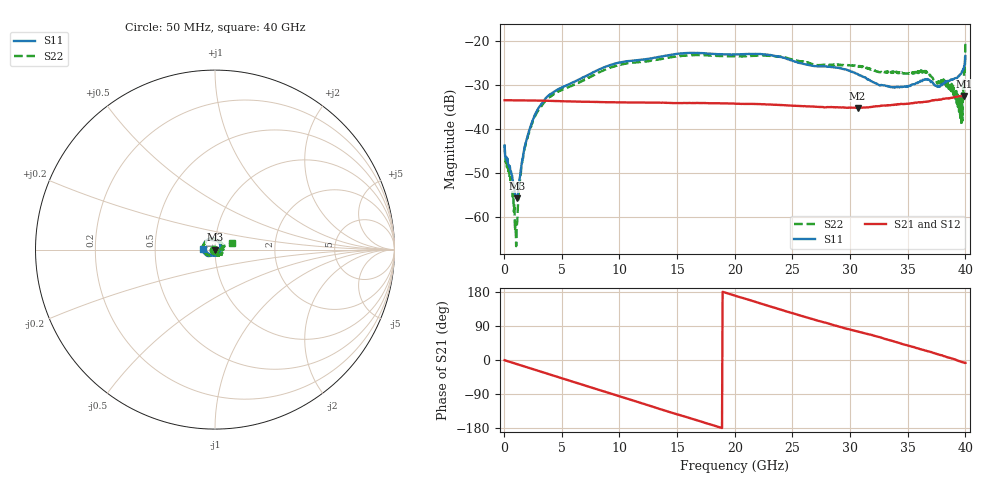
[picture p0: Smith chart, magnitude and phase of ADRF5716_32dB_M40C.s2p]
! Device: ADRF5716
! Description: 30GHz 2-Bit Digital Attenuator
! Frequency: 100 MHz – 30 GHz
! Ports:
! ATTIN  = Port 1
! ATTOUT = Port 2
! State: 32 dB Attenuation selected
! Supply Voltage:
! VDD  =  +3.30 Volts
! VSS  =  -3.30 Volts
! Control Voltages:
! D5 = 0V, D6 = 3.3V
! Temperature = -40 C
! Data: Data was collected using a calibrated network analyzer.
!  The reference plane is the package pins of ADRF5716 switch.
! Note: Analog Devices supplies this data as a sample of measured data for this product.
!  Your particular data for this product may vary.
!  Analog Devices reserves the right to change this data at anytime
# HZ S DB R 50
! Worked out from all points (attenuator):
!   800 points, 50 MHz to 40 GHz, reference 50 ohm
!   highest |S21| = -32.51 dB at 39.9 GHz (marker M1); lowest = -35.2 dB at 30.65 GHz (marker M2)
!   lowest |S11| = -55.8 dB at 1.1 GHz (marker M3), VSWR 1.00, Z = 49.9 - j0.119 ohm
!   |S11| at or under -10 dB: start of sweep to end of sweep
!   |S22| runs from -66.7 to -19.9 dB; largest |S21 - S12| = 0
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5e7  -43.81 -140.6  -33.48 -0.6  -33.48 -0.6  -43.64 -138.2
6e8  -49.65 177.3  -33.49 -5.9  -33.49 -5.9  -50.97 168.2
9.5e8  -54.84 -154.8  -33.51 -9.3  -33.51 -9.3  -63.17 -178.2
1.1e9  -55.77 -132.8  -33.52 -10.7  -33.52 -10.7  -62.14 -112.1
1.5e9  -48.55 -79.6  -33.53 -14.5  -33.53 -14.5  -48.74 -63.2
1.7e9  -45.37 -75.1  -33.53 -16.4  -33.53 -16.4  -45.27 -63.5
2.7e9  -36.64 -83.6  -33.55 -26.0  -33.55 -26.0  -36.96 -79.7
3.9e9  -32.30 -102.0  -33.62 -37.6  -33.62 -37.6  -32.87 -101.0
6.75e9  -28.42 -121.9  -33.81 -64.6  -33.81 -64.6  -29.17 -124.0
9.65e9  -25.12 -141.2  -33.95 -92.4  -33.95 -92.4  -25.67 -144.2
1.34e10  -23.63 -163.8  -34.03 -128.1  -34.03 -128.1  -24.20 -169.7
2.005e10  -23.06 154.0  -34.26 169.5  -34.26 169.5  -23.48 143.9
2.67e10  -25.64 101.0  -34.92 108.3  -34.92 108.3  -25.31 82.9
3.065e10  -27.55 49.6  -35.22 75.2  -35.22 75.2  -25.67 37.8
3.335e10  -30.34 10.3  -34.61 52.9  -34.61 52.9  -27.16 3.3
3.665e10  -28.82 -61.2  -33.77 23.8  -33.77 23.8  -26.99 -46.7
3.76e10  -30.45 -86.0  -33.39 15.1  -33.39 15.1  -29.29 -59.8
3.87e10  -28.85 -111.9  -32.97 5.3  -32.97 5.3  -29.54 -69.3
3.955e10  -27.64 -145.8  -32.61 -3.8  -32.61 -3.8  -37.72 -65.8
3.975e10  -26.89 -157.2  -32.59 -5.7  -32.59 -5.7  -38.13 -13.5
3.99e10  -25.63 -170.1  -32.51 -6.9  -32.51 -6.9  -25.43 16.6
4e10  -23.43 176.7  -32.61 -7.7  -32.61 -7.7  -19.89 20.8
